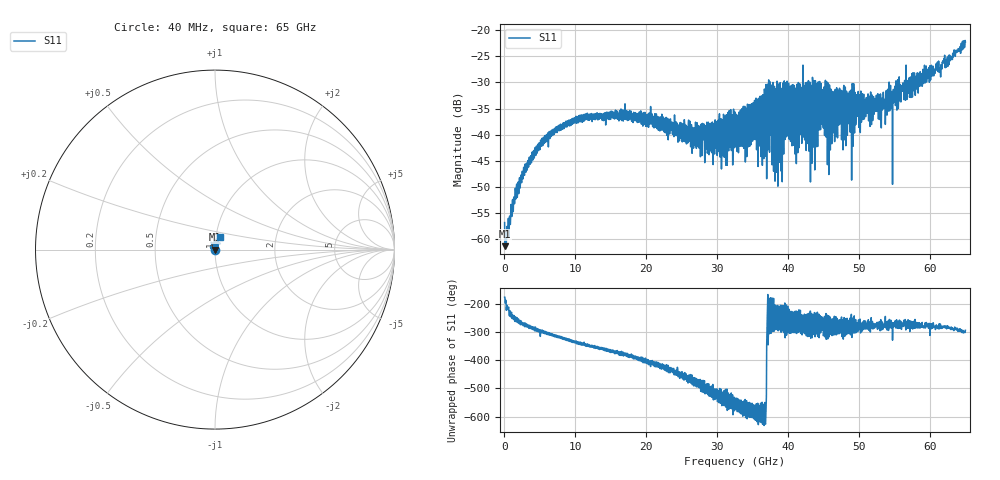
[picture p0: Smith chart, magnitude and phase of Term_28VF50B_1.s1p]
! Created Tue Jul 15 17:40:19 2008
# hz S ma R 50
! 2 Port Network Data from blockName block
! freq  magS11  angS11
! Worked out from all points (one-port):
!   1601 points, 40 MHz to 65 GHz, reference 50 ohm
!   lowest |S11| = -61.3 dB at 80.6 MHz (marker M1), VSWR 1.00, Z = 49.9 - j0.00814 ohm
!   |S11| at or under -10 dB: start of sweep to end of sweep
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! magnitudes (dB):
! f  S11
! 40 MHz  -56.8
! 80.6 MHz  -61.3
! 405.4 MHz  -59.1
! 1.461 GHz  -53.1
! 3.044 GHz  -47.2
! 5.44 GHz  -42.0
! 8.16 GHz  -38.4
! 16.28 GHz  -35.4
! 24.4 GHz  -38.0
! 28.54 GHz  -37.6
! 32.52 GHz  -35.7
! 36.46 GHz  -32.3
! 37.39 GHz  -43.4
! 38.29 GHz  -31.2
! 39.58 GHz  -40.9
! 40.64 GHz  -31.2
! 42.35 GHz  -41.0
! 43.48 GHz  -29.6
! 43.56 GHz  -42.4
! 44.54 GHz  -37.4
! 45.88 GHz  -31.4
! 48.76 GHz  -39.5
! 53.43 GHz  -31.9
! 54.12 GHz  -35.5
! 54.85 GHz  -31.3
! 55.17 GHz  -34.0
! 56.88 GHz  -31.6
! 65 GHz  -22.3
